| TEXAS INSTRUMENTS INCORPORATED
| Standard Linear and Logic Group
| IBIS Model of SN74ACT245
| OCTAL BUS TRANSCEIVERS WITH 3-STATE OUTPUTS
| This file contains package information for the following:
|  PDIP 20-pin (N) package as [Component] ACT245_N
|  SSOP 20-pin (DB) package as [Component] ACT245_DB
|  SOIC 20-pin (DW) package as [Component] ACT245_DW
|  SOP 20-pin (NS) package as [Component] ACT245_NS
|  TSSOP 20-pin (PW) package as [Component] ACT245_PW
| This device can be powered at the following Vccs:
|  5 volt Vcc
| This file provides unique models under the [Model Selector] for each Vcc.
| For operation at a specific Vcc, select the appropriate model after each
| [Model Selector] keyword.
[IBIS Ver]   3.2
[Comment char]  |_char
[File Name]   sn74act245.ibs
[File Rev]   1.1 | a_die
[Date]   September 4, 2003
[Source]   Data created from TI-SPICE simulations at TI-SLL.
[Notes]   The following is an IBIS list for the ACT245.
   Please contact sllibis@ti.com with questions and
   comments concerning SLL IBIS models.
   This IBIS model is created from a BA (back annotated netlist)
[Disclaimer] Property of Texas Instruments Incorporated.  Unauthorized
   reproduction and/or distribution is strictly prohibited.
   This product is protected under copyright law.
   Created  2003, (C) Copyright  2003, Texas Instruments
   Incorporated, All Rights Reserved
   UNLESS THERE IS A SIGNED, WRITTEN AGREEMENT TO THE
   CONTRARY, TEXAS INSTRUMENTS (TI) IS PROVIDING THE IBIS
   MODELS  AND WITHOUT ANY WARRANTY, EXPRESSED OR
   IMPLIED.  TI assumes no liability for:
   1) the accuracy of the IBIS models provided to your
   company;
   2) the proper functioning of these IBIS Models in your
   design or for any resulting applications; or
   3) infringement of patents, copyrights or intellectual
   property rights resulting from your use of these IBIS
   models.
   TI provides IBIS Models as a service to our customers.
   You and your company shall not distribute, sell or give
   these models to anyone else without prior written
   permission from TI.
   TI reserves the right to make changes to our products or
   to discontinue any semiconductor product or service
   without notice, and advises our customers to obtain the
   latest version of relevant information to verify, before
   placing orders, that the information being relied on is
   current.
   Please be aware that your receipt and use of the IBIS
   information provided shall serve as acceptance of these
   terms and conditions.  If you do not accept these terms,
   you should return or destroy the IBIS models and any
   other accompanying information immediately.
| Component ACT245_N 20-pin PDIP
[Component]   ACT245_N
[Manufacturer]   Texas Instruments, Inc.
[Package]
|   typ   min   max
R_pkg   4.300e-02   3.800e-02   5.000e-02
L_pkg   7.384e-09   4.680e-09   1.032e-08
C_pkg   5.100e-13   2.310e-13   8.210e-13
[Pin]   signal_name   model_name   R_pin   L_pin   C_pin
1   DIR   ACT245_DIR   4.200e-02   9.427e-09   8.100e-13
2   A1   ACT245_IO   4.600e-02   8.544e-09   4.560e-13
3   A2   ACT245_IO   4.800e-02   7.163e-09   4.350e-13
4   A3   ACT245_IO   4.000e-02   4.825e-09   2.610e-13
5   A4   ACT245_IO   4.000e-02   5.284e-09   6.480e-13
6   A5   ACT245_IO   4.000e-02   4.686e-09   2.320e-13
7   A6   ACT245_IO   4.000e-02   6.359e-09   4.890e-13
8   A7   ACT245_IO   3.800e-02   7.982e-09   4.750e-13
9   A8   ACT245_IO   4.300e-02   9.403e-09   4.750e-13
10   GND   GND   5.000e-02   1.032e-08   8.050e-13
11   B8   ACT245_IO   5.000e-02   1.028e-08   8.100e-13
12   B7   ACT245_IO   4.300e-02   9.383e-09   4.770e-13
13   B6   ACT245_IO   3.800e-02   7.978e-09   4.760e-13
14   B5   ACT245_IO   4.000e-02   6.302e-09   4.920e-13
15   B4   ACT245_IO   4.000e-02   4.680e-09   2.310e-13
16   B3   ACT245_IO   4.000e-02   5.284e-09   6.480e-13
17   B2   ACT245_IO   4.000e-02   4.822e-09   2.610e-13
18   B1   ACT245_IO   4.700e-02   7.118e-09   4.390e-13
19   NOE   ACT245_NOE   4.600e-02   8.492e-09   4.610e-13
20   VCC   POWER   4.300e-02   9.348e-09   8.210e-13
| Component ACT245_DB 20-pin SSOP
[Component]   ACT245_DB
[Manufacturer]   Texas Instruments, Inc.
[Package]
|   typ   min   max
R_pkg   4.000e-02   3.500e-02   5.100e-02
L_pkg   3.495e-09   3.035e-09   4.314e-09
C_pkg   4.200e-13   3.460e-13   5.020e-13
[Pin]   signal_name   model_name   R_pin   L_pin   C_pin
1   DIR   ACT245_DIR   4.900e-02   4.310e-09   5.020e-13
2   A1   ACT245_IO   4.800e-02   3.903e-09   4.870e-13
3   A2   ACT245_IO   3.500e-02   3.189e-09   3.960e-13
4   A3   ACT245_IO   3.500e-02   3.036e-09   3.470e-13
5   A4   ACT245_IO   3.500e-02   3.035e-09   3.670e-13
6   A5   ACT245_IO   3.500e-02   3.035e-09   3.670e-13
7   A6   ACT245_IO   3.500e-02   3.036e-09   3.470e-13
8   A7   ACT245_IO   3.500e-02   3.189e-09   3.970e-13
9   A8   ACT245_IO   4.700e-02   3.899e-09   4.880e-13
10   GND   GND   5.100e-02   4.314e-09   5.000e-13
11   B8   ACT245_IO   5.100e-02   4.314e-09   5.000e-13
12   B7   ACT245_IO   4.700e-02   3.899e-09   4.880e-13
13   B6   ACT245_IO   3.500e-02   3.189e-09   3.970e-13
14   B5   ACT245_IO   3.500e-02   3.036e-09   3.460e-13
15   B4   ACT245_IO   3.500e-02   3.035e-09   3.670e-13
16   B3   ACT245_IO   3.500e-02   3.035e-09   3.670e-13
17   B2   ACT245_IO   3.500e-02   3.036e-09   3.460e-13
18   B1   ACT245_IO   3.500e-02   3.189e-09   3.970e-13
19   NOE   ACT245_NOE   4.700e-02   3.899e-09   4.880e-13
20   VCC   POWER   5.100e-02   4.314e-09   5.020e-13
| Component ACT245_DW 20-pin SOIC
[Component]   ACT245_DW
[Manufacturer]   Texas Instruments, Inc.
[Package]
|   typ   min   max
R_pkg   3.800e-02   3.300e-02   4.500e-02
L_pkg   5.012e-09   4.110e-09   6.349e-09
C_pkg   7.170e-13   5.300e-13   8.680e-13
[Pin]   signal_name   model_name   R_pin   L_pin   C_pin
1   DIR   ACT245_DIR   4.200e-02   6.336e-09   8.650e-13
2   A1   ACT245_IO   4.300e-02   5.542e-09   8.670e-13
3   A2   ACT245_IO   3.400e-02   4.714e-09   7.320e-13
4   A3   ACT245_IO   3.400e-02   4.377e-09   5.910e-13
5   A4   ACT245_IO   3.600e-02   4.130e-09   5.330e-13
6   A5   ACT245_IO   3.500e-02   4.111e-09   5.300e-13
7   A6   ACT245_IO   3.400e-02   4.284e-09   5.830e-13
8   A7   ACT245_IO   3.400e-02   4.634e-09   7.260e-13
9   A8   ACT245_IO   4.000e-02   5.518e-09   8.650e-13
10   GND   GND   4.300e-02   6.349e-09   8.660e-13
11   B8   ACT245_IO   4.100e-02   6.281e-09   8.610e-13
12   B7   ACT245_IO   4.500e-02   5.561e-09   8.680e-13
13   B6   ACT245_IO   3.300e-02   4.778e-09   7.420e-13
14   B5   ACT245_IO   3.500e-02   4.414e-09   5.960e-13
15   B4   ACT245_IO   3.500e-02   4.110e-09   5.330e-13
16   B3   ACT245_IO   3.600e-02   4.130e-09   5.330e-13
17   B2   ACT245_IO   3.400e-02   4.377e-09   5.910e-13
18   B1   ACT245_IO   3.400e-02   4.714e-09   7.310e-13
19   NOE   ACT245_NOE   4.300e-02   5.569e-09   8.680e-13
20   VCC   POWER   4.200e-02   6.308e-09   8.640e-13
| Component ACT245_NS 20-pin SOP
[Component]   ACT245_NS
[Manufacturer]   Texas Instruments, Inc.
[Package]
|   typ   min   max
R_pkg   4.400e-02   2.900e-02   5.800e-02
L_pkg   3.666e-09   2.317e-09   5.115e-09
C_pkg   5.480e-13   3.160e-13   7.250e-13
[Pin]   signal_name   model_name   R_pin   L_pin   C_pin
1   DIR   ACT245_DIR   5.800e-02   5.115e-09   7.250e-13
2   A1   ACT245_IO   5.300e-02   4.591e-09   7.240e-13
3   A2   ACT245_IO   4.900e-02   3.754e-09   5.720e-13
4   A3   ACT245_IO   2.900e-02   2.549e-09   3.880e-13
5   A4   ACT245_IO   3.100e-02   2.317e-09   3.160e-13
6   A5   ACT245_IO   3.100e-02   2.317e-09   3.160e-13
7   A6   ACT245_IO   2.900e-02   2.556e-09   3.990e-13
8   A7   ACT245_IO   4.900e-02   3.754e-09   5.790e-13
9   A8   ACT245_IO   5.300e-02   4.591e-09   7.240e-13
10   GND   GND   5.800e-02   5.115e-09   7.250e-13
11   B8   ACT245_IO   5.800e-02   5.115e-09   7.250e-13
12   B7   ACT245_IO   5.300e-02   4.591e-09   7.240e-13
13   B6   ACT245_IO   4.900e-02   3.754e-09   5.790e-13
14   B5   ACT245_IO   2.900e-02   2.557e-09   3.990e-13
15   B4   ACT245_IO   3.100e-02   2.317e-09   3.160e-13
16   B3   ACT245_IO   3.100e-02   2.317e-09   3.160e-13
17   B2   ACT245_IO   2.900e-02   2.557e-09   3.990e-13
18   B1   ACT245_IO   4.900e-02   3.754e-09   5.790e-13
19   NOE   ACT245_NOE   5.300e-02   4.591e-09   7.240e-13
20   VCC   POWER   5.800e-02   5.115e-09   7.250e-13
| Component ACT245_PW 20-pin TSSOP
[Component]   ACT245_PW
[Manufacturer]   Texas Instruments, Inc.
[Package]
|   typ   min   max
R_pkg   5.000e-02   4.200e-02   6.000e-02
L_pkg   2.802e-09   2.248e-09   3.553e-09
C_pkg   3.170e-13   2.020e-13   4.430e-13
[Pin]   signal_name   model_name   R_pin   L_pin   C_pin
1   DIR   ACT245_DIR   5.500e-02   3.461e-09   4.400e-13
2   A1   ACT245_IO   5.500e-02   3.150e-09   4.010e-13
3   A2   ACT245_IO   4.200e-02   2.619e-09   3.020e-13
4   A3   ACT245_IO   4.500e-02   2.273e-09   2.020e-13
5   A4   ACT245_IO   4.500e-02   2.248e-09   2.240e-13
6   A5   ACT245_IO   4.500e-02   2.273e-09   2.260e-13
7   A6   ACT245_IO   4.400e-02   2.323e-09   2.050e-13
8   A7   ACT245_IO   4.600e-02   2.704e-09   3.070e-13
9   A8   ACT245_IO   6.000e-02   3.265e-09   4.110e-13
10   GND   GND   5.700e-02   3.506e-09   4.360e-13
11   B8   ACT245_IO   5.800e-02   3.553e-09   4.370e-13
12   B7   ACT245_IO   5.800e-02   3.193e-09   4.050e-13
13   B6   ACT245_IO   4.200e-02   2.704e-09   3.110e-13
14   B5   ACT245_IO   4.600e-02   2.392e-09   2.100e-13
15   B4   ACT245_IO   4.700e-02   2.334e-09   2.290e-13
16   B3   ACT245_IO   4.700e-02   2.300e-09   2.270e-13
17   B2   ACT245_IO   4.700e-02   2.349e-09   2.070e-13
18   B1   ACT245_IO   4.500e-02   2.677e-09   3.060e-13
19   NOE   ACT245_NOE   6.000e-02   3.235e-09   4.060e-13
20   VCC   POWER   5.600e-02   3.487e-09   4.430e-13
| Models and submodels in the file (3): ACT245_DIR (Input), ACT245_NOE (Input), ACT245_IO (I/O)
